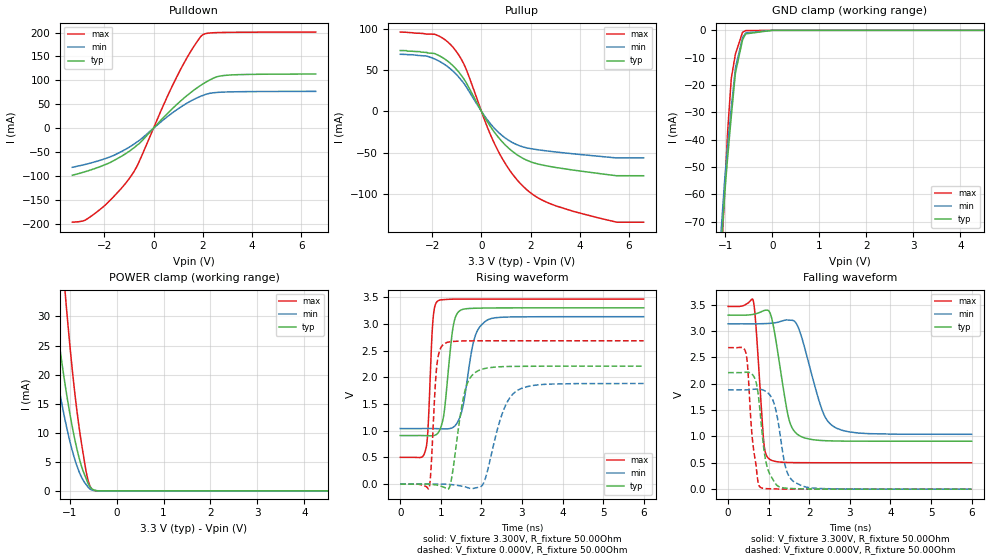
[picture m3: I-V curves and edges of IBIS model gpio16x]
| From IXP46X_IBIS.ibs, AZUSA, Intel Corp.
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[Model]   gpio16x
Model_type   I/O
Vinl = 800.000mV
Vinh = 2.000V
Vmeas = 1.500V
Cref = 0.000F
|   typ   min   max
C_comp   3.000pF   2.700pF   3.300pF
[Voltage Range]   3.300V   3.135V   3.465V
[Temperature Range]   25.0   110.0   -40.0
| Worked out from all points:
|   slope of the pulldown table from 0 to 0.495 V, typ, clamps not added: 18.3 ohm
|   slope of the pullup table from 0 to 0.495 V, typ, clamps not added: 20.7 ohm
|   POWER clamp passes 1 mA (typ) near -0.59 V on its own axis
|   falling waveform, V_fixture 3.300V, R_fixture 50.00Ohm: 20-80 % time 303ps typ, 464ps min, 152ps max; typ from 3.3 V to 0.909 V
|   rising waveform, V_fixture 3.300V, R_fixture 50.00Ohm: 20-80 % time 189ps typ, 278ps min, 100ps max; typ from 0.909 V to 3.3 V
|   rising waveform, V_fixture 0.000V, R_fixture 50.00Ohm: 20-80 % time 273ps typ, 426ps min, 116ps max; typ from 0 V to 2.21 V
|   falling waveform, V_fixture 0.000V, R_fixture 50.00Ohm: 20-80 % time 210ps typ, 256ps min, 175ps max; typ from 2.21 V to 0 V
[Pulldown]
|   Voltage   I(typ)   I(min)   I(max)
-3.3V     -98.37mA   -81.69mA   -196.5mA
-2.775V   -90.85mA   -75.66mA   -192.1mA
-2.295V   -82.72mA   -69.02mA   -174.8mA
-1.595V   -67.13mA   -56.33mA   -141.8mA
-920mV    -45.86mA   -37.53mA   -100.6mA
-610mV    -33.33mA   -26.76mA   -72.86mA
940mV     49.3mA     38.37mA    106.8mA
1.535V    75.39mA    57.37mA    162.3mA
1.99V     91.91mA    68.2mA     195mA
2.545V    107mA      74.63mA    199.8mA
2.875V    110.3mA    75.57mA    200.2mA
6.595V    113.3mA    77.04mA    200.9mA
[GND Clamp]
|   Voltage   I(typ)   I(min)   I(max)
-3.3V     -1.837A    -1.782A    -2.189A
-1.105V   -83.54mA   -76.82mA   -91.9mA
-1.015V   -60.22mA   -54.85mA   -58.27mA
-990mV    -54.49mA   -49.76mA   -50.02mA
-950mV    -46.11mA   -42mA      -36.59mA
-875mV    -31.64mA   -28.64mA   -17.74mA
-785mV    -15.52mA   -13.65mA   -8.609mA
-635mV    -3.528mA   -2.728mA   -731.7uA
-575mV    -1.509mA   -1.11mA    -135.3uA
0V        -56.84nA   -17.58nA   -565.5pA
6.595V    0A         0A         0A
[Pullup]
|   Voltage   I(typ)   I(min)   I(max)
-3.3V     73.53mA    68.99mA    95.85mA
-1.9V     69.78mA    63.29mA    93.19mA
-1.065V   52.36mA    45.95mA    74.19mA
-630mV    35.21mA    30.23mA    51.58mA
215mV     -11.3mA    -9.309mA   -17.3mA
695mV     -31.7mA    -25.52mA   -48.9mA
1.25V     -48.26mA   -37.63mA   -75.53mA
1.945V    -60.5mA    -44.86mA   -97.43mA
2.78V     -66.75mA   -48.4mA    -111.6mA
3.83V     -71.55mA   -51.73mA   -121.8mA
5.5V      -77.95mA   -56.45mA   -134.2mA
6.595V    -77.99mA   -56.45mA   -134.2mA
[POWER Clamp]
|   Voltage   I(typ)   I(min)   I(max)
-3.3V     221.1mA    178.3mA    361mA
-1.53V    46.58mA    33.69mA    83.8mA
-1.35V    33.69mA    23.73mA    61.53mA
-1.11V    19.11mA    12.77mA    35.67mA
-1.08V    17.53mA    11.61mA    32.8mA
-930mV    10.52mA    6.586mA    19.92mA
-800mV    5.804mA    3.373mA    11.15mA
-640mV    2mA        1.037mA    3.043mA
-595mV    1.12mA     542.7uA    1.52mA
-540mV    479.4uA    207uA      465.4uA
-395mV    31.37uA    12.42uA    6.173uA
6.595V    0A         0A         0A
[Ramp]
R_load = 50.00Ohm
|   typ   min   max
dV/dt_r   1.326V/272.290ps   1.130V/424.484ps   1.610V/115.937ps
dV/dt_f   1.435V/302.265ps   1.257V/463.036ps   1.779V/151.848ps
[Falling Waveform]
V_fixture = 3.300V
V_fixture_min = 3.135V
V_fixture_max = 3.465V
R_fixture = 50.00Ohm
|   Time   V(typ)   V(min)   V(max)
0s        3.3V       3.135V     3.465V
620ps     3.314V     3.134V     3.571V
690ps     3.327V     3.134V     3.041V
880ps     3.385V     3.138V     874.8mV
1.03ns    3.345V     3.144V     563mV
1.49ns    1.351V     3.205V     505.2mV
1.73ns    1.028V     3.063V     502.9mV
2.31ns    922.4mV    1.513V     500.9mV
2.63ns    913.6mV    1.173V     500.8mV
6ns       909mV      1.04V      500.8mV
[Rising Waveform]
V_fixture = 3.300V
V_fixture_min = 3.135V
V_fixture_max = 3.465V
R_fixture = 50.00Ohm
|   Time   V(typ)   V(min)   V(max)
0s        909mV      1.04V      500.8mV
630ps     907.1mV    1.041V     655.8mV
810ps     906.5mV    1.04V      3.104V
930ps     956.4mV    1.037V     3.432V
1.08ns    1.329V     1.034V     3.455V
1.31ns    2.975V     1.067V     3.463V
1.47ns    3.248V     1.252V     3.464V
1.84ns    3.293V     2.757V     3.465V
2.17ns    3.298V     3.081V     3.465V
6ns       3.3V       3.135V     3.465V
[Rising Waveform]
V_fixture = 0.000V
V_fixture_min = 0.000V
V_fixture_max = 0.000V
R_fixture = 50.00Ohm
|   Time   V(typ)   V(min)   V(max)
0s        743.2nV    272.8nV    -2.577nV
710ps     -682.9uV   279.9uV    -77.4mV
900ps     -18.27mV   793.8uV    2.203V
1.1ns     -66.41mV   -1.026mV   2.636V
1.25ns    47.22mV    -8.448mV   2.668V
1.59ns    1.73V      -50.31mV   2.682V
1.86ns    2.096V     -71.27mV   2.683V
2.08ns    2.164V     65.54mV    2.683V
2.86ns    2.205V     1.74V      2.684V
6ns       2.209V     1.883V     2.684V
[Falling Waveform]
V_fixture = 0.000V
V_fixture_min = 0.000V
V_fixture_max = 0.000V
R_fixture = 50.00Ohm
|   Time   V(typ)   V(min)   V(max)
0s        2.209V     1.883V     2.684V
440ps     2.217V     1.882V     2.574V
610ps     2.161V     1.893V     859.3mV
710ps     1.952V     1.898V     292mV
800ps     1.359V     1.893V     31.71mV
900ps     652.9mV    1.866V     12.57mV
1.04ns    264.1mV    1.773V     6.739mV
1.45ns    17.56mV    329.3mV    1.094mV
1.83ns    5.547mV    60.16mV    115.5uV
6ns       743.2nV    272.8nV    -2.577nV
